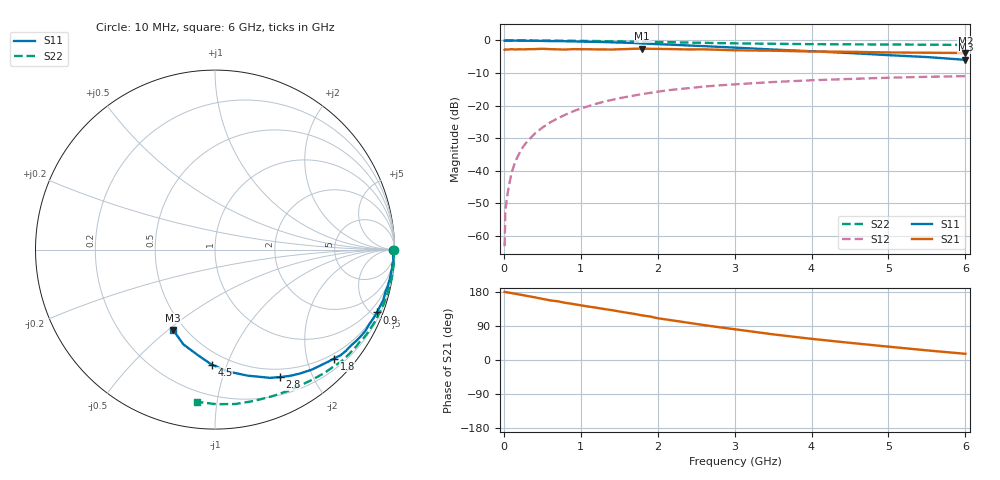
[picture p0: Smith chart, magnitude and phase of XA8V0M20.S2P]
! SIEMENS Discrete & RF Semiconductors
! BFY180
! Si NPN RF Bipolar Junction Transistor in MICRO-X
! VCE = 8 V  IC = 0.2 mA
! Common Emitter S-Parameters:  May  1997
# GHz  S  MA  R  50
!  f  S11  S21  S12  S22
! GHz  MAG  ANG  MAG  ANG  MAG  ANG  MAG  ANG
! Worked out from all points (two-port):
!   36 points, 10 MHz to 6 GHz, reference 50 ohm
!   highest |S21| = -2.51 dB at 1.8 GHz (marker M1); lowest = -3.8 dB at 6 GHz (marker M2)
!   |S21| within 3 dB of the highest: start of sweep to end of sweep
!   lowest |S11| = -5.9 dB at 6 GHz (marker M3), VSWR 3.04, Z = 21.6 - j26 ohm
!   |S11| at or under -10 dB: nowhere
!   |S22| runs from -1.4 to 0.0 dB; largest |S21 - S12| = 0.74
!   S11 on the Smith chart (normalised r, x): 10 MHz: open; 900 MHz: 0.48, -5.30; 1.8 GHz: 0.40, -2.52; 2.8 GHz: 0.40, -1.56; 4.5 GHz: 0.41, -0.88; 6 GHz: 0.43, -0.52
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0.01  0.9922 -0.1  0.718 179.6  0.0007 97.2  0.9986 -0.1
0.02  0.9898 -0.4  0.729 179.3  0.0025 97.7  0.9999 -0.4
0.05  0.9939 -1.0  0.725 178.3  0.0046 84.4  0.9989 -0.9
0.1  0.993 -2.4  0.736 176.6  0.0094 90.8  0.9964 -2.0
0.15  0.9968 -3.7  0.727 174.7  0.014 87.6  0.9999 -3.0
0.2  0.9909 -4.6  0.733 172.9  0.0184 85.6  0.9989 -4.0
0.25  0.9936 -5.9  0.73 171.2  0.0234 85.4  0.9999 -5.0
0.3  0.9895 -7.0  0.734 169.2  0.0278 84.3  0.9983 -5.8
0.4  0.9874 -9.6  0.737 165.5  0.0371 82.3  0.9985 -7.8
0.5  0.9839 -12.0  0.745 161.4  0.046 79.6  0.9968 -9.8
0.7  0.979 -16.6  0.73 154.9  0.064 75.2  0.9924 -13.7
0.9  0.9677 -21.2  0.736 147.8  0.0819 71.1  0.988 -17.6
1.1  0.9546 -25.9  0.734 141.0  0.0982 67.1  0.9809 -21.4
1.3  0.9447 -30.8  0.729 134.7  0.115 62.7  0.975 -25.3
1.8  0.8985 -42.5  0.749 117.6  0.1509 53.2  0.9539 -34.5
2.2  0.8594 -51.1  0.737 104.3  0.176 45.6  0.9399 -41.6
2.6  0.8188 -59.2  0.731 92.2  0.196 38.9  0.9199 -48.0
2.8  0.7971 -63.0  0.719 86.5  0.2046 35.7  0.9105 -51.1
3.5  0.7255 -75.5  0.696 67.7  0.2305 25.5  0.8895 -61.3
4.5  0.6408 -91.7  0.669 45.3  0.2568 12.9  0.8709 -75.4
5.5  0.5565 -108.5  0.648 25.4  0.2771 1.1  0.8612 -89.7
6  0.5045 -117.6  0.642 16.3  0.2834 -4.9  0.8535 -96.9
